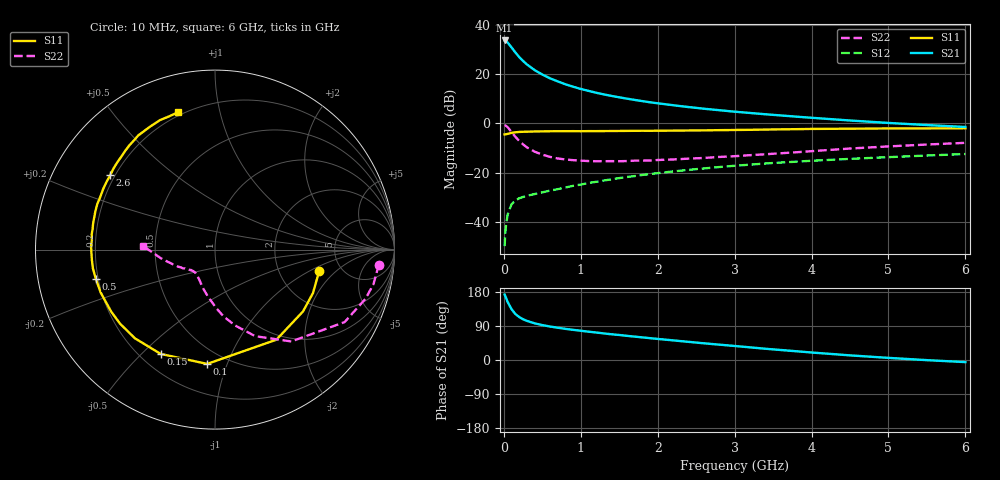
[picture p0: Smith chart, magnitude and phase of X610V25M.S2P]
! SIEMENS Small Signal Semiconductors
! BFP193W
! Si NPN RF Bipolar Junction Transistor in SOT343
! VCE = 10 V  IC = 25 mA
! Common Emitter S-Parameters:  April 1994
# GHz  S  MA  R  50
!  f  S11  S21  S12  S22
! GHz  MAG  ANG  MAG  ANG  MAG  ANG  MAG  ANG
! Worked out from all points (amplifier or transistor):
!   40 points, 10 MHz to 6 GHz, reference 50 ohm
!   highest |S21| = 33.6 dB at 10 MHz (marker M1)
!   |S21| within 3 dB of that: start of sweep to 104.4 MHz
!   unconditionally stable (mu >= 1): 957.8 MHz to 4.859 GHz
!   at 200 MHz: K = 0.38, MSG = 28.7 dB, |S12| = -30.5 dB
!   at 1.5 GHz: K = 1.10, MAG = 14.5 dB, |S12| = -22.3 dB
!   at 6 GHz: K = 0.96, MSG = 5.5 dB, |S12| = -12.5 dB
!   S11 on the Smith chart (normalised r, x): 10 MHz: 3.40, -1.26; 100 MHz: 0.40, -0.85; 150 MHz: 0.28, -0.57; 500 MHz: 0.19, -0.12; 2.6 GHz: 0.18, +0.31; 6 GHz: 0.18, +0.75
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0.01  0.5926 -11.7  47.86 172.8  0.0032 70.8  0.9166 -5.2
0.02  0.5972 -23.9  47.37 168.1  0.0063 73.0  0.9037 -12.3
0.03  0.5993 -35.1  46.26 163.0  0.009 72.9  0.8821 -18.1
0.05  0.6075 -55.7  43.26 152.9  0.0141 65.3  0.8275 -29.2
0.1  0.6383 -93.9  34.59 134.0  0.0226 51.7  0.6653 -50.3
0.15  0.6553 -117.5  27.3 121.3  0.0273 44.5  0.5317 -65.1
0.2  0.6659 -132.1  22.01 113.3  0.03 41.8  0.437 -75.2
0.25  0.671 -142.1  18.38 107.5  0.0319 40.1  0.3731 -83.0
0.3  0.6739 -149.2  15.6 103.2  0.0336 39.7  0.3232 -89.1
0.4  0.6804 -159.4  12 96.8  0.0366 40.5  0.265 -98.5
0.5  0.6838 -166.3  9.73 92.1  0.0395 42.7  0.2304 -105.9
0.6  0.6882 -171.2  8.16 88.3  0.0429 44.7  0.2077 -111.7
0.8  0.689 -178.8  6.183 82.2  0.0497 48.3  0.1838 -119.8
1.1  0.6921 172.8  4.543 74.7  0.0612 51.7  0.1708 -128.3
1.3  0.694 168.3  3.846 70.1  0.0688 53.1  0.1697 -131.8
1.6  0.6998 162.3  3.157 63.7  0.081 53.7  0.1708 -135.8
2.2  0.7089 151.3  2.321 51.8  0.1052 52.8  0.184 -143.1
2.6  0.716 144.7  1.973 44.1  0.121 51.2  0.1974 -147.8
3.2  0.7353 135.2  1.616 33.4  0.1444 47.9  0.2249 -154.8
4.5  0.7747 117.9  1.137 12.2  0.1892 39.6  0.3067 -171.1
5.5  0.7848 109.3  0.918 -0.4  0.2213 33.7  0.3697 -179.8
6  0.792 105.2  0.84 -5.6  0.2375 31.1  0.4005 176.9
